| IBIS file stm32f7x3_ufbga144.ibs
[IBIS ver] 4.2
[File name] stm32f7x3_ufbga144.ibs
[File Rev] 1.1
[Date]  21-12-2016
[Source] Data Created at STMicroelectronics
[Notes]  File originated from ELDO simulations.
[Disclaimer]  This information is for modeling purpose only and is
   not guaranted.
   The information is subject to change without notice.
[Copyright] Copyright 2017 STMicroelectronics Inc.
|   Component stm32f7x3_ufbga144
[Component] stm32f7x3_ufbga144
[Manufacturer] STMicroelectronics
[Package]
| variable   typ   min   max
R_pkg   0.0   0.0   0.0
L_pkg   0.0H   0.0H   0.0H
C_pkg   0.0F   0.0F   0.0F
[Pin]  signal_name   model_name   R_pin   L_pin   C_pin
A1 PC13 io8p_arwsudq_ft_v33
A10 PA15 io8p_arsudq_ft
A11 PA14 io8p_arsudq_ft
A12 PA13 io8p_arsudq_ft
A2 PE3 io8p_arsudq_ft
A3 PE2 io8p_arsudq_ft
A4 PE1 io8p_arsudq_ft
A5 PE0 io8p_arsudq_ft
A6 PB4 io8p_arsudq_ft
A7 PB3 io8p_arsudq_ft
A8 PD6 io8p_arsudq_ft
A9 PD7 io8p_arsudq_ft
B1 PC14-OSC32_IN io8p_arwsudq_ft_v33
B10 PC11 io8p_arsudq_ft
B11 PC10 io8p_arsudq_ft
B12 PA12 io8usb_lsfs_otg_ft
B2 PE4 io8p_arsudq_ft
B3 PE5 io8p_arsudq_ft
B4 PE6 io8p_arsudq_ft
B5 PB9 io8p_arsudq_i2c_ft
B6 PB5 io8p_ar3wsudq_ft
B7 PG15 io8p_arsudq_ft
B8 PG12 io8p_arsudq_ft
B9 PD5 io8p_arsudq_ft
C1 PC15-OSC32_OUT io8p_arwsudq_ft
C10 PC12 io8p_arsudq_ft
C11 VDDUSB power
C12 PA11 io8usb_lsfs_otg_ft
C2 VBAT power
C3 PF0 io8p_arsudq_i2c_ft
C4 PF1 io8p_arsudq_i2c_ft
C5 PB8 io8p_arsudq_i2c_ft
C6 PB6 io8p_arsudq_i2c_ft
C7 PG14 io8p_arsudq_ft
C8 PG11 io8p_arsudq_ft
C9 PD4 io8p_arsudq_ft
D1 PH0-OSC_IN io8p_arsudq_ft
D10 PD1 io8p_arsudq_ft
D11 PA10 io8usb_id_otg_ft
D12 PA9 io8usb_vbus_otg_ft
D2 VSS gnd
D3 VDD power
D4 PF2 io8p_arsudq_ft
D5 BOOT0 vpp_test_hv
D6 PB7 io8p_arsudq_i2c_ft
D7 PG13 io8p_arsudq_ft
D8 PG10 io8p_arsudq_ft
D9 PD3 io8p_arsudq_ft
E1 PH1-OSC_OUT io8p_arsudq_ft
E10 PD0 io8p_arsudq_ft
E11 PC9 io8p_arsudq_i2c_ft
E12 PA8 io8p_arsudq_i2c_ft
E2 PF3 io8p_arwsudq_ft
E3 PF4 io8p_arwsudq_ft
E4 PF5 io8p_arwsudq_ft
E5 PDR_ON_PAD gnd
E6 VSS gnd
E7 VSS gnd
E8 PG9 io8p_arsudq_ft
E9 PD2 io8p_arsudq_ft
F1 NRST ioreset_ft_v33
F10 VDD power
F11 PC8 io8p_arsudq_ft
F12 PC7 io8p_arsudq_ft
F2 PF7 io8p_arwsudq_ft
F3 PF6 io8p_arwsudq_ft
F4 VDD power
F5 VDD power
F6 VDD power
F7 VDDSDMMC power
F8 VDD power
F9 VDD power
G1 PF10 io8p_arwsudq_ft
G10 VSS gnd
G11 PG8 io8p_arsudq_ft
G12 PC6 io8p_arsudq_ft
G2 PF9 io8p_arwsudq_ft
G3 PF8 io8p_arwsudq_ft
G4 VSS gnd
G5 VDD power
G6 VDD power
G7 VDD power
G8 VSS gnd
G9 VCAP_2 power
H1 PC0 io8p_ar3wsudq_ft
H10 VDD12OTGHS power
H11 OTG_HS_REXT gnd
H12 PG5 io8p_arsudq_ft
H2 PC1 io8p_ar3wsudq_ft_v33
H3 PC2 io8p_ar3wsudq_ft
H4 PC3 io8p_ar3wsudq_ft
H5 BYPASS_REG gnd
H6 VSS gnd
H7 VCAP_1 power
H8 PE11 io8p_arsudq_ft
H9 PD11 io8p_arsudq_ft
J1 VSSA gnd
J10 PG4 io8p_arsudq_ft
J11 PG3 io8p_arsudq_ft
J12 PG2 io8p_arsudq_ft
J2 PA0 io8p_ar3wsudq_ft_v33
J3 PA4 io8p_ar3wsudq_ft
J4 PC4 io8p_ar3wsudq_ft
J5 PB2 io8p_ar3wsudq_ft
J6 PG1 io8p_arsudq_ft
J7 PE10 io8p_arsudq_ft
J8 PE12 io8p_arsudq_ft
J9 PD10 io8p_arsudq_ft
K1 VREF- gnd
K10 PD13 io8p_arsudq_ft
K11 PD14 io8p_arsudq_ft
K12 PD15 io8p_arsudq_ft
K2 PA1 io8p_ar3wsudq_ft
K3 PA5 io8p_ar3wsudq_ft
K4 PC5 io8p_ar3wsudq_ft
K5 PF13 io8p_arsudq_ft
K6 PG0 io8p_arsudq_ft
K7 PE9 io8p_arsudq_ft
K8 PE13 io8p_arsudq_ft
K9 PD9 io8p_arsudq_ft
L1 VREF+ power
L10 PD12 io8p_arsudq_ft
L11 PB14 io8p_arsudq_ft
L12 PB15 io8p_arsudq_ft
L2 PA2 io8p_ar3wsudq_ft_v33
L3 PA6 io8p_ar3wsudq_ft
L4 PB0 io8p_ar3wsudq_ft
L5 PF12 io8p_arsudq_ft
L6 PF15 io8p_arsudq_ft
L7 PE8 io8p_arsudq_ft
L8 PE14 io8p_arsudq_ft
L9 PD8 io8p_arsudq_ft
M1 VDDA power
M10 PB11 io8p_arsudq_i2c_ft
M11 PB12 io8usb_id_otg_ft
M12 PB13 io8usb_vbus_otg_ft
M2 PA3 io8p_ar3wsudq_ft
M3 PA7 io8p_ar3wsudq_ft
M4 PB1 io8p_ar3wsudq_ft
M5 PF11 io8p_arsudq_ft
M6 PF14 io8p_arsudq_ft
M7 PE7 io8p_arsudq_ft
M8 PE15 io8p_ar3wsudq_ft
M9 PB10 io8p_arsudq_i2c_ft
[Diff Pin]   inv_pin   vdiff   tdelay_typ  tdelay_min  tdelay_max
B12   C12   NA   NA   NA   NA
[Model Selector] io8p_ar3wsudq_ft
io8p00_ar3wsudq_ft_pd_lv  "SPEED00 1P8V, PD=40kOhm"
io8p00_ar3wsudq_ft_pu_lv  "SPEED00 1P8V, PU=40kOhm"
io8p00_ar3wsudq_ft_lv  "SPEED00 1P8V"
io8p01_ar3wsudq_ft_pd_lv  "SPEED01 1P8V, PD=40kOhm"
io8p01_ar3wsudq_ft_pu_lv  "SPEED01 1P8V, PU=40kOhm"
io8p01_ar3wsudq_ft_lv  "SPEED01 1P8V"
io8p10_ar3wsudq_ft_pd_lv  "SPEED10 1P8V, PD=40kOhm"
io8p10_ar3wsudq_ft_pu_lv  "SPEED10 1P8V, PU=40kOhm"
io8p10_ar3wsudq_ft_lv  "SPEED10 1P8V"
io8p11_ar3wsudq_ft_pd_lv  "SPEED11 1P8V, PD=40kOhm"
io8p11_ar3wsudq_ft_pu_lv  "SPEED11 1P8V, PU=40kOhm"
io8p11_ar3wsudq_ft_lv  "SPEED11 1P8V"
io8p00_ar3wsudq_ft_pd  "SPEED00, PD=40kOhm"
io8p00_ar3wsudq_ft_pu  "SPEED00, PU=40kOhm"
io8p00_ar3wsudq_ft  "SPEED00"
io8p01_ar3wsudq_ft_pd  "SPEED01, PD=40kOhm"
io8p01_ar3wsudq_ft_pu  "SPEED01, PU=40kOhm"
io8p01_ar3wsudq_ft  "SPEED01"
io8p10_ar3wsudq_ft_pd  "SPEED10, PD=40kOhm"
io8p10_ar3wsudq_ft_pu  "SPEED10, PU=40kOhm"
io8p10_ar3wsudq_ft  "SPEED10"
io8p11_ar3wsudq_ft_pd  "SPEED11, PD=40kOhm"
io8p11_ar3wsudq_ft_pu  "SPEED11, PU=40kOhm"
io8p11_ar3wsudq_ft  "SPEED11"
[Model Selector] io8p_ar3wsudq_ft_v33
io8p00_ar3wsudq_ft_v33_pd_lv  "SPEED00 1P8V, PD=40kOhm"
io8p00_ar3wsudq_ft_v33_pu_lv  "SPEED00 1P8V, PU=40kOhm"
io8p00_ar3wsudq_ft_v33_lv  "SPEED00 1P8V"
io8p01_ar3wsudq_ft_v33_pd_lv  "SPEED01 1P8V, PD=40kOhm"
io8p01_ar3wsudq_ft_v33_pu_lv  "SPEED01 1P8V, PU=40kOhm"
io8p01_ar3wsudq_ft_v33_lv  "SPEED01 1P8V"
io8p10_ar3wsudq_ft_v33_pd_lv  "SPEED10 1P8V, PD=40kOhm"
io8p10_ar3wsudq_ft_v33_pu_lv  "SPEED10 1P8V, PU=40kOhm"
io8p10_ar3wsudq_ft_v33_lv  "SPEED10 1P8V"
io8p11_ar3wsudq_ft_v33_pd_lv  "SPEED11 1P8V, PD=40kOhm"
io8p11_ar3wsudq_ft_v33_pu_lv  "SPEED11 1P8V, PU=40kOhm"
io8p11_ar3wsudq_ft_v33_lv  "SPEED11 1P8V"
io8p00_ar3wsudq_ft_v33_pd  "SPEED00, PD=40kOhm"
io8p00_ar3wsudq_ft_v33_pu  "SPEED00, PU=40kOhm"
io8p00_ar3wsudq_ft_v33  "SPEED00"
io8p01_ar3wsudq_ft_v33_pd  "SPEED01, PD=40kOhm"
io8p01_ar3wsudq_ft_v33_pu  "SPEED01, PU=40kOhm"
io8p01_ar3wsudq_ft_v33  "SPEED01"
io8p10_ar3wsudq_ft_v33_pd  "SPEED10, PD=40kOhm"
io8p10_ar3wsudq_ft_v33_pu  "SPEED10, PU=40kOhm"
io8p10_ar3wsudq_ft_v33  "SPEED10"
io8p11_ar3wsudq_ft_v33_pd  "SPEED11, PD=40kOhm"
io8p11_ar3wsudq_ft_v33_pu  "SPEED11, PU=40kOhm"
io8p11_ar3wsudq_ft_v33  "SPEED11"
[Model Selector] io8p_arsudq_ft
io8p00_arsudq_ft_pd_lv  "SPEED00 1P8V, PD=40kOhm"
io8p00_arsudq_ft_pu_lv  "SPEED00 1P8V, PU=40kOhm"
io8p00_arsudq_ft_lv  "SPEED00 1P8V"
io8p01_arsudq_ft_pd_lv  "SPEED01 1P8V, PD=40kOhm"
io8p01_arsudq_ft_pu_lv  "SPEED01 1P8V, PU=40kOhm"
io8p01_arsudq_ft_lv  "SPEED01 1P8V"
io8p10_arsudq_ft_pd_lv  "SPEED10 1P8V, PD=40kOhm"
io8p10_arsudq_ft_pu_lv  "SPEED10 1P8V, PU=40kOhm"
io8p10_arsudq_ft_lv  "SPEED10 1P8V"
io8p11_arsudq_ft_pd_lv  "SPEED11 1P8V, PD=40kOhm"
io8p11_arsudq_ft_pu_lv  "SPEED11 1P8V, PU=40kOhm"
io8p11_arsudq_ft_lv  "SPEED11 1P8V"
io8p00_arsudq_ft_pd  "SPEED00, PD=40kOhm"
io8p00_arsudq_ft_pu  "SPEED00, PU=40kOhm"
io8p00_arsudq_ft  "SPEED00"
io8p01_arsudq_ft_pd  "SPEED01, PD=40kOhm"
io8p01_arsudq_ft_pu  "SPEED01, PU=40kOhm"
io8p01_arsudq_ft  "SPEED01"
io8p10_arsudq_ft_pd  "SPEED10, PD=40kOhm"
io8p10_arsudq_ft_pu  "SPEED10, PU=40kOhm"
io8p10_arsudq_ft  "SPEED10"
io8p11_arsudq_ft_pd  "SPEED11, PD=40kOhm"
io8p11_arsudq_ft_pu  "SPEED11, PU=40kOhm"
io8p11_arsudq_ft  "SPEED11"
[Model Selector] io8p_arsudq_i2c_ft
io8prog_1v8_i2c_pd  "5V Tol GPIO 1.8V range i2c functionality with pull down"
io8prog_1v8_i2c_pu  "5V Tol GPIO 1.8V range i2c functionality with pull up"
io8prog_1v8_i2c  "5V Tol GPIO 1.8V range i2c functionality"
io8prog_3v3_i2c_pd  "5V Tol GPIO 3.3V range i2c functionality with pull down"
io8prog_3v3_i2c_pu  "5V Tol GPIO 3.3V range i2c functionality with pull up"
io8prog_3v3_i2c  "5V Tol GPIO 3.3V range i2c functionality"
io8prog_1v8_pd_00  "5V Tol GPIO 1.8V range with pd speed 00"
io8prog_1v8_pu_00  "5V Tol GPIO 1.8V range with pu speed 00"
io8prog_1v8_00  "5V Tol GPIO 1.8V range speed 00"
io8prog_3v3_pd_00  "5V Tol GPIO 3.3V range with pd speed 00"
io8prog_3v3_pu_00  "5V Tol GPIO 3.3V range with pu speed 00"
io8prog_3v3_00  "5V Tol GPIO 3.3V range speed 00"
io8prog_1v8_pd_01  "5V Tol GPIO 1.8V range with pd speed 01"
io8prog_1v8_pu_01  "5V Tol GPIO 1.8V range with pu speed 01"
io8prog_1v8_01  "5V Tol GPIO 1.8V range speed 01"
io8prog_3v3_pd_01  "5V Tol GPIO 3.3V range with pd speed 01"
io8prog_3v3_pu_01  "5V Tol GPIO 3.3V range with pu speed 01"
io8prog_3v3_01  "5V Tol GPIO 3.3V range speed 01"
io8prog_1v8_pd_10  "5V Tol GPIO 1.8V range with pd speed 10"
io8prog_1v8_pu_10  "5V Tol GPIO 1.8V range with pu speed 10"
io8prog_1v8_10  "5V Tol GPIO 1.8V range speed 10"
io8prog_3v3_pd_10  "5V Tol GPIO 3.3V range with pd speed 10"
io8prog_3v3_pu_10  "5V Tol GPIO 3.3V range with pu speed 10"
io8prog_3v3_10  "5V Tol GPIO 3.3V range speed 10"
io8prog_1v8_pd_11  "5V Tol GPIO 1.8V range with pd speed 11"
io8prog_1v8_pu_11  "5V Tol GPIO 1.8V range with pu speed 11"
io8prog_1v8_11  "5V Tol GPIO 1.8V range speed 11"
io8prog_3v3_pd_11  "5V Tol GPIO 3.3V range with pd speed 11"
io8prog_3v3_pu_11  "5V Tol GPIO 3.3V range with pu speed 11"
io8prog_3v3_11  "5V Tol GPIO 3.3V range speed 11"
[Model Selector] io8p_arwsudq_ft
io8p00_arwsudq_ft_pd_lv  "SPEED00 1P8V, PD=40kOhm"
io8p00_arwsudq_ft_pu_lv  "SPEED00 1P8V, PU=40kOhm"
io8p00_arwsudq_ft_lv  "SPEED00 1P8V"
io8p01_arwsudq_ft_pd_lv  "SPEED01 1P8V, PD=40kOhm"
io8p01_arwsudq_ft_pu_lv  "SPEED01 1P8V, PU=40kOhm"
io8p01_arwsudq_ft_lv  "SPEED01 1P8V"
io8p10_arwsudq_ft_pd_lv  "SPEED10 1P8V, PD=40kOhm"
io8p10_arwsudq_ft_pu_lv  "SPEED10 1P8V, PU=40kOhm"
io8p10_arwsudq_ft_lv  "SPEED10 1P8V"
io8p11_arwsudq_ft_pd_lv  "SPEED11 1P8V, PD=40kOhm"
io8p11_arwsudq_ft_pu_lv  "SPEED11 1P8V, PU=40kOhm"
io8p11_arwsudq_ft_lv  "SPEED11 1P8V"
io8p00_arwsudq_ft_pd  "SPEED00, PD=40kOhm"
io8p00_arwsudq_ft_pu  "SPEED00, PU=40kOhm"
io8p00_arwsudq_ft  "SPEED00"
io8p01_arwsudq_ft_pd  "SPEED01, PD=40kOhm"
io8p01_arwsudq_ft_pu  "SPEED01, PU=40kOhm"
io8p01_arwsudq_ft  "SPEED01"
io8p10_arwsudq_ft_pd  "SPEED10, PD=40kOhm"
io8p10_arwsudq_ft_pu  "SPEED10, PU=40kOhm"
io8p10_arwsudq_ft  "SPEED10"
io8p11_arwsudq_ft_pd  "SPEED11, PD=40kOhm"
io8p11_arwsudq_ft_pu  "SPEED11, PU=40kOhm"
io8p11_arwsudq_ft  "SPEED11"
[Model Selector] io8p_arwsudq_ft_v33
io8p00_arwsudq_ft_v33_pd_lv  "SPEED00 1P8V, PD=40kOhm"
io8p00_arwsudq_ft_v33_pu_lv  "SPEED00 1P8V, PU=40kOhm"
io8p00_arwsudq_ft_v33_lv  "SPEED00 1P8V"
io8p01_arwsudq_ft_v33_pd_lv  "SPEED01 1P8V, PD=40kOhm"
io8p01_arwsudq_ft_v33_pu_lv  "SPEED01 1P8V, PU=40kOhm"
io8p01_arwsudq_ft_v33_lv  "SPEED01 1P8V"
io8p10_arwsudq_ft_v33_pd_lv  "SPEED10 1P8V, PD=40kOhm"
io8p10_arwsudq_ft_v33_pu_lv  "SPEED10 1P8V, PU=40kOhm"
io8p10_arwsudq_ft_v33_lv  "SPEED10 1P8V"
io8p11_arwsudq_ft_v33_pd_lv  "SPEED11 1P8V, PD=40kOhm"
io8p11_arwsudq_ft_v33_pu_lv  "SPEED11 1P8V, PU=40kOhm"
io8p11_arwsudq_ft_v33_lv  "SPEED11 1P8V"
io8p00_arwsudq_ft_v33_pd  "SPEED00, PD=40kOhm"
io8p00_arwsudq_ft_v33_pu  "SPEED00, PU=40kOhm"
io8p00_arwsudq_ft_v33  "SPEED00"
io8p01_arwsudq_ft_v33_pd  "SPEED01, PD=40kOhm"
io8p01_arwsudq_ft_v33_pu  "SPEED01, PU=40kOhm"
io8p01_arwsudq_ft_v33  "SPEED01"
io8p10_arwsudq_ft_v33_pd  "SPEED10, PD=40kOhm"
io8p10_arwsudq_ft_v33_pu  "SPEED10, PU=40kOhm"
io8p10_arwsudq_ft_v33  "SPEED10"
io8p11_arwsudq_ft_v33_pd  "SPEED11, PD=40kOhm"
io8p11_arwsudq_ft_v33_pu  "SPEED11, PU=40kOhm"
io8p11_arwsudq_ft_v33  "SPEED11"
[Model Selector] io8usb_id_otg_ft
io8p00_id_otg_ft_pd_lv  "SPEED00 1P8V, PD=14kOhm"
io8p00_id_otg_ft_pu_lv  "SPEED00 1P8V, PU=14kOhm"
io8p00_id_otg_ft_lv  "SPEED00 1P8V"
io8p01_id_otg_ft_pd_lv  "SPEED01 1P8V, PD=14kOhm"
io8p01_id_otg_ft_pu_lv  "SPEED01 1P8V, PU=14kOhm"
io8p01_id_otg_ft_lv  "SPEED01 1P8V"
io8p10_id_otg_ft_pd_lv  "SPEED10 1P8V, PD=14kOhm"
io8p10_id_otg_ft_pu_lv  "SPEED10 1P8V, PU=14kOhm"
io8p10_id_otg_ft_lv  "SPEED10 1P8V"
io8p11_id_otg_ft_pd_lv  "SPEED11 1P8V, PD=14kOhm"
io8p11_id_otg_ft_pu_lv  "SPEED11 1P8V, PU=14kOhm"
io8p11_id_otg_ft_lv  "SPEED11 1P8V"
io8p00_id_otg_ft_pd  "SPEED00, PD=14kOhm"
io8p00_id_otg_ft_pu  "SPEED00, PU=14kOhm"
io8p00_id_otg_ft  "SPEED00"
io8p01_id_otg_ft_pd  "SPEED01, PD=14kOhm"
io8p01_id_otg_ft_pu  "SPEED01, PU=14kOhm"
io8p01_id_otg_ft  "SPEED01"
io8p10_id_otg_ft_pd  "SPEED10, PD=14kOhm"
io8p10_id_otg_ft_pu  "SPEED10, PU=14kOhm"
io8p10_id_otg_ft  "SPEED10"
io8p11_id_otg_ft_pd  "SPEED11, PD=14kOhm"
io8p11_id_otg_ft_pu  "SPEED11, PU=14kOhm"
io8p11_id_otg_ft  "SPEED11"
[Model Selector] io8usb_lsfs_otg_ft
io8usb_ls_otg_ft_dpdn_pd  "LS USB DP/DN IO + PD=20kOhm"
io8usb_ls_otg_ft_dpdn_pupu2  "LS USB DP/DN IO + PU/PU2=2.2kOhm"
io8usb_ls_otg_ft_dpdn_pu2  "LS USB DP/DN IO + PU2=1.2kOhm"
io8usb_ls_otg_ft_dpdn_pu  "LS USB DP/DN IO + PU=1.2kOhm"
io8usb_ls_otg_ft_dpdn  "LS USB DP/DN IO"
io8usb_fs_otg_ft_dpdn_pd  "HS USB DP/DN IO + PD=20kOhm"
io8usb_fs_otg_ft_dpdn_pupu2  "HS USB DP/DN IO + PU/PU2=2.2kOhm"
io8usb_fs_otg_ft_dpdn_pu2  "HS USB DP/DN IO + PU2=1.2kOhm"
io8usb_fs_otg_ft_dpdn_pu  "HS USB DP/DN IO + PU=1.2kOhm"
io8usb_fs_otg_ft_dpdn  "HS USB DP/DN IO"
io8p00_lsfs_otg_ft_pd_lv  "SPEED00 1P8V, PD=40kOhm"
io8p00_lsfs_otg_ft_pu_lv  "SPEED00 1P8V, PU=40kOhm"
io8p00_lsfs_otg_ft_lv  "SPEED00 1P8V"
io8p01_lsfs_otg_ft_pd_lv  "SPEED01 1P8V, PD=40kOhm"
io8p01_lsfs_otg_ft_pu_lv  "SPEED01 1P8V, PU=40kOhm"
io8p01_lsfs_otg_ft_lv  "SPEED01 1P8V"
io8p10_lsfs_otg_ft_pd_lv  "SPEED10 1P8V, PD=40kOhm"
io8p10_lsfs_otg_ft_pu_lv  "SPEED10 1P8V, PU=40kOhm"
io8p10_lsfs_otg_ft_lv  "SPEED10 1P8V"
io8p11_lsfs_otg_ft_pd_lv  "SPEED11 1P8V, PD=40kOhm"
io8p11_lsfs_otg_ft_pu_lv  "SPEED11 1P8V, PU=40kOhm"
io8p11_lsfs_otg_ft_lv  "SPEED11 1P8V"
io8p00_lsfs_otg_ft_pd  "SPEED00, PD=40kOhm"
io8p00_lsfs_otg_ft_pu  "SPEED00, PU=40kOhm"
io8p00_lsfs_otg_ft  "SPEED00"
io8p01_lsfs_otg_ft_pd  "SPEED01, PD=40kOhm"
io8p01_lsfs_otg_ft_pu  "SPEED01, PU=40kOhm"
io8p01_lsfs_otg_ft  "SPEED01"
io8p10_lsfs_otg_ft_pd  "SPEED10, PD=40kOhm"
io8p10_lsfs_otg_ft_pu  "SPEED10, PU=40kOhm"
io8p10_lsfs_otg_ft  "SPEED10"
io8p11_lsfs_otg_ft_pd  "SPEED11, PD=40kOhm"
io8p11_lsfs_otg_ft_pu  "SPEED11, PU=40kOhm"
io8p11_lsfs_otg_ft  "SPEED11"
[Model Selector] io8usb_vbus_otg_ft
io8psenb_vbus_otg_ft  "VBUS PULSE, SENSE VB"
io8psenab_vbus_otg_ft  "VBUS PULSE, SENSE VA and VB"
io8psena_vbus_otg_ft  "VBUS PULSE, SENSE VA"
io8psen_vbus_otg_ft  "VBUS PULSE"
io8p00_vbus_otg_ft_pd_lv  "SPEED00 1P8V, PD=40kOhm"
io8p00_vbus_otg_ft_pu_lv  "SPEED00 1P8V, PU=40kOhm"
io8p00_vbus_otg_ft_lv  "SPEED00 1P8V"
io8p01_vbus_otg_ft_pd_lv  "SPEED01 1P8V, PD=40kOhm"
io8p01_vbus_otg_ft_pu_lv  "SPEED01 1P8V, PU=40kOhm"
io8p01_vbus_otg_ft_lv  "SPEED01 1P8V"
io8p10_vbus_otg_ft_pd_lv  "SPEED10 1P8V, PD=40kOhm"
io8p10_vbus_otg_ft_pu_lv  "SPEED10 1P8V, PU=40kOhm"
io8p10_vbus_otg_ft_lv  "SPEED10 1P8V"
io8p11_vbus_otg_ft_pd_lv  "SPEED11 1P8V, PD=40kOhm"
io8p11_vbus_otg_ft_pu_lv  "SPEED11 1P8V, PU=40kOhm"
io8p11_vbus_otg_ft_lv  "SPEED11 1P8V"
io8p00_vbus_otg_ft_pd  "SPEED00, PD=40kOhm"
io8p00_vbus_otg_ft_pu  "SPEED00, PU=40kOhm"
io8p00_vbus_otg_ft  "SPEED00"
io8p01_vbus_otg_ft_pd  "SPEED01, PD=40kOhm"
io8p01_vbus_otg_ft_pu  "SPEED01, PU=40kOhm"
io8p01_vbus_otg_ft  "SPEED01"
io8p10_vbus_otg_ft_pd  "SPEED10, PD=40kOhm"
io8p10_vbus_otg_ft_pu  "SPEED10, PU=40kOhm"
io8p10_vbus_otg_ft  "SPEED10"
io8p11_vbus_otg_ft_pd  "SPEED11, PD=40kOhm"
io8p11_vbus_otg_ft_pu  "SPEED11, PU=40kOhm"
io8p11_vbus_otg_ft  "SPEED11"
[Model Selector] ioreset_ft_v33
ioreset_ft_v33_pu_lv  "IORESET 1P8V + PU=40kOhm"
ioreset_ft_v33_nopu_lv  "IORESET 1P8V"
ioreset_ft_v33_pu  "IORESET + PU=40kOhm"
ioreset_ft_v33_nopu  "IORESET"
[Model Selector] vpp_test_hv
vpp_test_hv_2p4  "Input Buffer 1P8V"
vpp_test_hv_3p3  "Input Buffer"
| Models and submodels in the file (242): io8p00_ar3wsudq_ft_pd_lv (I/O), io8p00_ar3wsudq_ft_pu_lv (I/O), io8p00_ar3wsudq_ft_lv (I/O), io8p01_ar3wsudq_ft_pd_lv (I/O), io8p01_ar3wsudq_ft_pu_lv (I/O), io8p01_ar3wsudq_ft_lv (I/O), io8p10_ar3wsudq_ft_pd_lv (I/O), io8p10_ar3wsudq_ft_pu_lv (I/O), io8p10_ar3wsudq_ft_lv (I/O), io8p11_ar3wsudq_ft_pd_lv (I/O), io8p11_ar3wsudq_ft_pu_lv (I/O), io8p11_ar3wsudq_ft_lv (I/O), io8p00_ar3wsudq_ft_pd (I/O), io8p00_ar3wsudq_ft_pu (I/O), io8p00_ar3wsudq_ft (I/O), io8p01_ar3wsudq_ft_pd (I/O), io8p01_ar3wsudq_ft_pu (I/O), io8p01_ar3wsudq_ft (I/O), io8p10_ar3wsudq_ft_pd (I/O), io8p10_ar3wsudq_ft_pu (I/O), io8p10_ar3wsudq_ft (I/O), io8p11_ar3wsudq_ft_pd (I/O), io8p11_ar3wsudq_ft_pu (I/O), io8p11_ar3wsudq_ft (I/O), io8p00_ar3wsudq_ft_v33_pd_lv (I/O), io8p00_ar3wsudq_ft_v33_pu_lv (I/O), io8p00_ar3wsudq_ft_v33_lv (I/O), io8p01_ar3wsudq_ft_v33_pd_lv (I/O), io8p01_ar3wsudq_ft_v33_pu_lv (I/O), io8p01_ar3wsudq_ft_v33_lv (I/O), io8p10_ar3wsudq_ft_v33_pd_lv (I/O), io8p10_ar3wsudq_ft_v33_pu_lv (I/O), io8p10_ar3wsudq_ft_v33_lv (I/O), io8p11_ar3wsudq_ft_v33_pd_lv (I/O), io8p11_ar3wsudq_ft_v33_pu_lv (I/O), io8p11_ar3wsudq_ft_v33_lv (I/O), io8p00_ar3wsudq_ft_v33_pd (I/O), io8p00_ar3wsudq_ft_v33_pu (I/O), io8p00_ar3wsudq_ft_v33 (I/O), io8p01_ar3wsudq_ft_v33_pd (I/O), io8p01_ar3wsudq_ft_v33_pu (I/O), io8p01_ar3wsudq_ft_v33 (I/O), io8p10_ar3wsudq_ft_v33_pd (I/O), io8p10_ar3wsudq_ft_v33_pu (I/O), io8p10_ar3wsudq_ft_v33 (I/O), io8p11_ar3wsudq_ft_v33_pd (I/O), io8p11_ar3wsudq_ft_v33_pu (I/O), io8p11_ar3wsudq_ft_v33 (I/O), io8p00_arsudq_ft_pd_lv (I/O), io8p00_arsudq_ft_pu_lv (I/O), io8p00_arsudq_ft_lv (I/O), io8p01_arsudq_ft_pd_lv (I/O), io8p01_arsudq_ft_pu_lv (I/O), io8p01_arsudq_ft_lv (I/O), io8p10_arsudq_ft_pd_lv (I/O), io8p10_arsudq_ft_pu_lv (I/O), io8p10_arsudq_ft_lv (I/O), io8p11_arsudq_ft_pd_lv (I/O), io8p11_arsudq_ft_pu_lv (I/O), io8p11_arsudq_ft_lv (I/O), io8p00_arsudq_ft_pd (I/O), io8p00_arsudq_ft_pu (I/O), io8p00_arsudq_ft (I/O), io8p01_arsudq_ft_pd (I/O), io8p01_arsudq_ft_pu (I/O), io8p01_arsudq_ft (I/O), io8p10_arsudq_ft_pd (I/O), io8p10_arsudq_ft_pu (I/O), io8p10_arsudq_ft (I/O), io8p11_arsudq_ft_pd (I/O), io8p11_arsudq_ft_pu (I/O), io8p11_arsudq_ft (I/O), io8prog_1v8_i2c_pd (I/O), io8prog_1v8_i2c_pu (I/O), io8prog_1v8_i2c (I/O), io8prog_3v3_i2c_pd (I/O), io8prog_3v3_i2c_pu (I/O), io8prog_3v3_i2c (I/O), io8prog_1v8_pd_00 (I/O), io8prog_1v8_pu_00 (I/O)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
